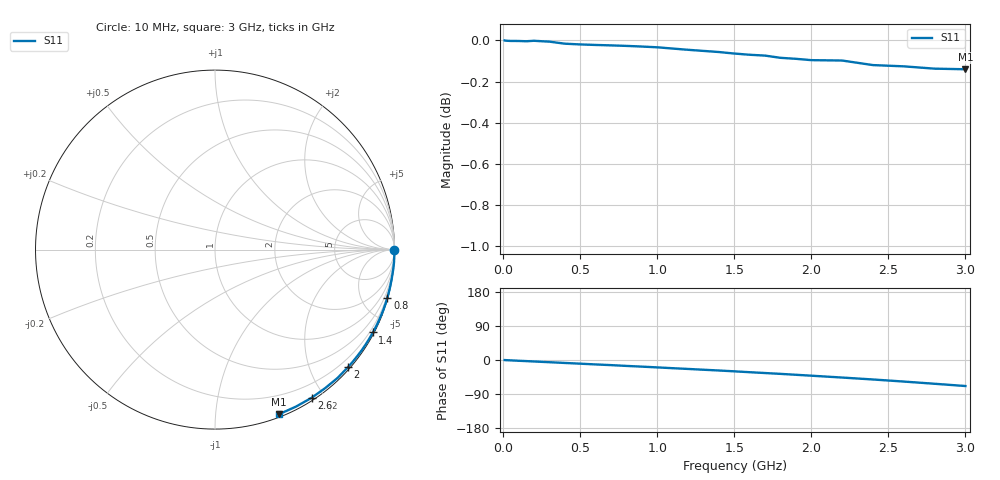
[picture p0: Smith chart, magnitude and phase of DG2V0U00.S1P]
! SIEMENS Small Signal Semiconductors
! BAV70
! Silicon Switching Diode in SOT23
! VR = 2 V
! S-Parameters:  May  1995
# GHz  S  MA  R  50
!  f  S11
! GHz  MAG  ANG
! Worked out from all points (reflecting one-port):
!   30 points, 10 MHz to 3 GHz, reference 50 ohm
!   lowest |S11| = -0.1 dB at 3 GHz (marker M1), VSWR 124.00, Z = 1.27 - j73.1 ohm
!   phase of S11 starts at -0 deg and turns -68 deg over the sweep
!   S11 on the Smith chart (normalised r, x): 10 MHz: open; 800 MHz: 0.08, -7.30; 1.4 GHz: 0.06, -4.06; 2 GHz: 0.04, -2.65; 2.6 GHz: 0.03, -1.85; 3 GHz: 0.03, -1.46
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0.01  1 -0.2
0.1  0.9997 -2.0
0.15  0.9995 -2.9
0.2  0.9998 -3.9
0.25  0.9996 -4.9
0.3  0.9993 -5.8
0.4  0.9982 -7.8
0.5  0.9978 -9.7
0.6  0.9975 -11.7
0.7  0.9972 -13.5
0.8  0.997 -15.6
0.9  0.9966 -17.5
1  0.9962 -19.5
1.1  0.9955 -21.6
1.2  0.9948 -23.6
1.3  0.9942 -25.7
1.4  0.9935 -27.7
1.5  0.9927 -29.9
1.6  0.992 -32.2
1.7  0.9916 -34.4
1.8  0.9903 -36.6
1.9  0.9898 -39.0
2  0.989 -41.4
2.2  0.9888 -46.3
2.4  0.9863 -51.4
2.6  0.9856 -56.9
2.8  0.9843 -62.7
3  0.984 -68.7
